PROGRAM IO_EXCHANGE
VAR
	WRITE_SINT			:	FB_EcCoESdoWrite	;
	sNetId              : 	T_AmsNetId := '10.4.6.84.7.1'; (* NetId of EtherCAT Master *)     
    nSlaveAddr_1        : 	UINT := 1003; (* Port Number of EtherCAT Slave *) 
	SDO_WRITE			:	STR_SDO	;
	WRITE_DATA_SINT		:	USINT;
	WRITE_EN_SINT		:	BOOL;
END_VAR

PLC_TO_UI();
UI_TO_PLC();

//************************HW-IO******************************************
//C02
		GV.NDI.	AV101_OPEN	:=	ECC.	CHAMBER_IN.		C02	[	1	];	//	AV101OPEN
		GV.NDI.	AV101_CLOSE	:=	ECC.	CHAMBER_IN.		C02	[	2	];	//	AV101CLOSE
		GV.NDI.	AV102_OPEN	:=	ECC.	CHAMBER_IN.		C02	[	3	];	//	AV102OPEN
	//	GV.NDI.	AV102_CLOSE	:=	ECC.	CHAMBER_IN.		C02	[	4	];	//	AV102CLOSE
	//	GV.NDI.	AV103_OPEN	:=									
	//	GV.NDI.	AV103_CLOSE	:=									
		GV.NDI.	AV104_OPEN	:=	ECC.	CHAMBER_IN.		C02	[	5	];	//	AV104OPEN
	//	GV.NDI.	AV104_CLOSE	:=	ECC.	CHAMBER_IN.		C02	[	6	];	//	AV104CLOSE
		GV.NDI.	AV105_OPEN	:=	ECC.	CHAMBER_IN.		C02	[	7	];	//	AV105OPEN
	//	GV.NDI.	AV105_CLOSE	:=	ECC.	CHAMBER_IN.		C02	[	8	];	//	AV105CLOSE
		GV.NDI.	AV106_OPEN	:=	ECC.	CHAMBER_IN.		C02	[	9	];	//	AV106OPEN
		GV.NDI.	AV106_CLOSE	:=	ECC.	CHAMBER_IN.		C02	[	10	];	//	AV106CLOSE
		GV.NDI.	CY1_OPEN	:=	ECC.	CHAMBER_IN.		C02	[	11	];	//	CY1 UP
		GV.NDI.	CY1_CLOSE	:=	ECC.	CHAMBER_IN.		C02	[	12	];	//	CY1 DOWN
		GV.NDI.	Lift_Pin_Middle1	:=	ECC.	CHAMBER_IN.		C02	[	13	];	//	CY1 Middle
		GV.NDI.	CY2_OPEN	:=	ECC.	CHAMBER_IN.		C02	[	14	];	//	CY2 UP						 
		GV.NDI.	CY2_CLOSE	:=	ECC.	CHAMBER_IN.		C02	[	15	];	//	CY2 DOWN
		GV.NDI.	Lift_Pin_Middle2	:=	ECC.	CHAMBER_IN.		C02	[	16	];	//	CY2 Middle								

//C03																											
		GV.NDI.	GV1_OPEN			:=	ECC.	CHAMBER_IN.		C03	[	1	];		//Slit Door Opened
		GV.NDI.	GV1_CLOSE			:=	ECC.	CHAMBER_IN.		C03	[	2	];		//Slit Door Closed
		GV.NDI.FL02B2				:=	ECC.	CHAMBER_IN.		C03	[	3	];		
		//							:=	ECC.	CHAMBER_IN.		C03	[	4	];		
		GV.NDI.FL03B2				:=	ECC.	CHAMBER_IN.		C03	[	5	];		
		//							:=	ECC.	CHAMBER_IN.		C03	[	6	];		
		GV.NDI.FL04B2				:=	ECC.	CHAMBER_IN.		C03	[	7	];		
		GV.NDI.Robot_Extend_TO_PM	:=	ECC.	CHAMBER_IN.		C03	[	8	];		//Robot Extend To PM
					//				:=	ECC.	CHAMBER_IN.		C03	[	9	];		
		GV.NDI.CDA_OK				:=	ECC.	CHAMBER_IN.		C03	[	10	];		
		GV.NDI.SYS_CDA_OK			:=	ECC.	CHAMBER_IN.		C03	[	11	];		//SYS CDA OK
		GV.NDI.SYS_N2_OK			:=	ECC.	CHAMBER_IN.		C03	[	12	];		//SYS N2 OK
		GV.NDI.TM_Lid_Closed		:=	ECC.	CHAMBER_IN.		C03	[	13	];		//TM Lid Closed
					//				:=	ECC.	CHAMBER_IN.		C03	[	14	];		
					//				:=	ECC.	CHAMBER_IN.		C03	[	15	];		//
					//				:=	ECC.	CHAMBER_IN.		C03	[	16	];		//

//C04
		GV.AI.	APC_Temp				:=			INT_TO_REAL(	ECC.	CHAMBER_IN.	C04	[	1	])/10;	//	SSR1	钟摆阀(E01)	TC01
		GV.AI.	Lid_Temp				:=			INT_TO_REAL(	ECC.	CHAMBER_IN.	C04	[	2	])/10;	//	SSR2	LID HEATER控温TC	(E02-E05) TC02
		GV.AI.	Lid_Temp_Monitor1		:=			INT_TO_REAL(	ECC.	CHAMBER_IN.	C04	[	3	])/10;	//	LID HEATER TC monitor	TC03
		GV.AI.	Lid_Temp_Monitor2		:=			INT_TO_REAL(	ECC.	CHAMBER_IN.	C04	[	4	])/10;	//	LID HEATER TC monitor	TC04
		GV.AI.	Chamber_Temp1			:=			INT_TO_REAL(	ECC.	CHAMBER_IN.	C04	[	5	])/10;	//	SSR3	CHAMBER HEATER 控温TC (E06,E07)	TC05
		GV.AI.	Chamber_Temp2			:=			INT_TO_REAL(	ECC.	CHAMBER_IN.	C04	[	6	])/10;	//	SSR4	CHAMBER HEATER 控温TC (E08,E09,E12,E13)	TC06
		GV.AI.	Chamber_Temp3			:=			INT_TO_REAL(	ECC.	CHAMBER_IN.	C04	[	7	])/10;	//	SSR5	CHAMBER HEATER 控温TC (E10,E11)			TC07
		GV.AI.	Stage_Temp1				:=			INT_TO_REAL(	ECC.	CHAMBER_IN.	C04	[	8	])/10;	//	CHILLER控温用(左侧内)	TC08

//C05		
		GV.AI.	Stage_Temp2				:=			INT_TO_REAL(	ECC.	CHAMBER_IN.	C05	[	1	])/10;	//	CHILLER控温用(左侧外)	TC09 
		GV.AI.	Stage_Temp3				:=			INT_TO_REAL(	ECC.	CHAMBER_IN.	C05	[	2	])/10;	//	CHILLER控温用(右侧内)	TC10
		GV.AI.	Stage_Temp4				:=			INT_TO_REAL(	ECC.	CHAMBER_IN.	C05	[	3	])/10;	//	CHILLER控温用(右侧外)	TC11
		GV.AI.	Chamber_Temp_Monitor	:=			INT_TO_REAL(	ECC.	CHAMBER_IN.	C05	[	4	])/10;	//	腔体底部监控用	TC12
		GV.AI.	Gate_Valve_Temp			:=			INT_TO_REAL(	ECC.	CHAMBER_IN.	C05	[	5	])/10;	//	SSR18	GATE VALVE控温用	E18 TC13
		GV.AI.	Gate_Valve_Temp_Monitor	:=			INT_TO_REAL(	ECC.	CHAMBER_IN.	C05	[	6	])/10;	//	GATE VALVE监控	TC14
										//			INT_TO_REAL(	ECC.	CHAMBER_IN.	C05	[	7	])/10;	//	
										//			INT_TO_REAL(	ECC.	CHAMBER_IN.	C05	[	8	])/10;	//	

//C06							
										//							ECC.	CHAMBER_IN.	C06	[	1	]);
										//							ECC.	CHAMBER_IN.	C06	[	2	]);
										//							ECC.	CHAMBER_IN.	C06	[	3	]);
										//							ECC.	CHAMBER_IN.	C06	[	4	]);

							
//C07											
		ECC.	CHAMBER_OUT.	C07	[	1	]	:=	TRUE;//GV_IL.TMP_PW_EN;//GV.TURBO_PUMP_POWER_ON							;	
		ECC.	CHAMBER_OUT.	C07	[	2	]	:=	GV_IL.HTR_APC_EN;//GV.PENDULUM_VALVE_HEATER_POWER_ON				;	
		ECC.	CHAMBER_OUT.	C07	[	3	]	:=	GV_IL.HTR_LID_EN;//GV.LID_HEATER_POWER_ON							;	
		ECC.	CHAMBER_OUT.	C07	[	4	]	:=	GV_IL.HTR_CHAMBER_EN;//GV.CHAMBER_HEATER_POWER_ON						;	
		ECC.	CHAMBER_OUT.	C07	[	5	]	:=	GV_IL.HTR_GAS_BOX_EN;//GV.IGS_HEATER_POWER_ON							;	
		ECC.	CHAMBER_OUT.	C07	[	6	]	:=	GV_IL.HTR_GAS_BOX_EN;//GV.TAPE_HEATER_POWER_ON							;	
		ECC.	CHAMBER_OUT.	C07	[	7	]	:=	GV_IL.HTR_FORLINE_EN;//GV.FORELINE_HEATER_POWER_ON						;	
		ECC.	CHAMBER_OUT.	C07	[	8	]	:=	GV_IL.HTR_GATE_VALVE_EN;//GV.GATE_VALVE_HEATER_POWER_ON					;	
	//	ECC.	CHAMBER_OUT.	C07	[	9	]	:=			;	
	//	ECC.	CHAMBER_OUT.	C07	[	10	]	:=			;	
	//	ECC.	CHAMBER_OUT.	C07	[	11	]	:=			;	
	//	ECC.	CHAMBER_OUT.	C07	[	12	]	:=			;	
		ECC.	CHAMBER_OUT.	C07	[	13	]	:=	GV.NDO.GV_Open_Enable		;	//Slit Door Open Enable
		ECC.	CHAMBER_OUT.	C07	[	14	]	:=	GV.NDO.GV_Close_Enable		;	//Slit Door Close Enable
		ECC.	CHAMBER_OUT.	C07	[	15	]	:=	GV.NDO.TM_Robot_Extend_Enable AND GV.NDI.CY1_OPEN AND GV.NDI.CY2_OPEN		;	//Robot Extend Enable
		ECC.	CHAMBER_OUT.	C07	[	16	]	;//:=			;	
												
//C08												
		ECC.	CHAMBER_OUT.	C08	[	1	]	:=	GV.LID_HEATER_SSR_ON[1]		;	//SSR02
	//	ECC.	CHAMBER_OUT.	C08	[	2	]	:=	GV.LID_HEATER_SSR_ON[2]		;	//SSR02
	//	ECC.	CHAMBER_OUT.	C08	[	3	]	:=	GV.LID_HEATER_SSR_ON[3]		;	//SSR02
	//	ECC.	CHAMBER_OUT.	C08	[	4	]	:=	GV.LID_HEATER_SSR_ON[4]		;	//SSR02
	//	ECC.	CHAMBER_OUT.	C08	[	5	]	:=								;	
	//	ECC.	CHAMBER_OUT.	C08	[	6	]	:=								;	
		ECC.	CHAMBER_OUT.	C08	[	7	]	:=	GV.CHAMBER_HEATER_SSR_ON[1]	;	//SSR03
		ECC.	CHAMBER_OUT.	C08	[	8	]	:=	GV.CHAMBER_HEATER_SSR_ON[2]	;	//SSR03
		ECC.	CHAMBER_OUT.	C08	[	9	]	:=	GV.CHAMBER_HEATER_SSR_ON[3]	;	//SSR04	
	//	ECC.	CHAMBER_OUT.	C08	[	10	]	:=	
		ECC.	CHAMBER_OUT.	C08	[	11	]	:=	GV.CHAMBER_HEATER_SSR_ON[4];	//SSR05
	//	ECC.	CHAMBER_OUT.	C08	[	12	]	:=	
		ECC.	CHAMBER_OUT.	C08	[	13	]	:=	
	//	ECC.	CHAMBER_OUT.	C08	[	14	]	:=	
	//	ECC.	CHAMBER_OUT.	C08	[	15	]	:=								;	
	//	ECC.	CHAMBER_OUT.	C08	[	16	]	:=								;	
												
//C09												
		ECC.	CHAMBER_OUT.	C09	[	1	]	:=	GV.FORELINE_HEATER_SSR_ON[1];	//SSR6	AV102 E33
		ECC.	CHAMBER_OUT.	C09	[	2	]	:=	GV.FORELINE_HEATER_SSR_ON[2];	//SSR7	AV101 E36
		ECC.	CHAMBER_OUT.	C09	[	3	]	:=	GV.FORELINE_HEATER_SSR_ON[3];	//SSR8	AV106	E38
		ECC.	CHAMBER_OUT.	C09	[	4	]	:=	GV.FORELINE_HEATER_SSR_ON[4];	//SSR9	BA01	
	//	ECC.	CHAMBER_OUT.	C09	[	5	]	:=								;	
	//	ECC.	CHAMBER_OUT.	C09	[	6	]	:=								;	
		ECC.	CHAMBER_OUT.	C09	[	7	]	:=	GV.GATE_VALVE_SSR_ON		;	//SSR18
	//	ECC.	CHAMBER_OUT.	C09	[	8	]	:=								;	
		ECC.	CHAMBER_OUT.	C09	[	9	]	:=	GV.PEN_VALVE_HEATER_SSR_ON	;	//SSR01
	//	ECC.	CHAMBER_OUT.	C09	[	10	]	:=								;	
		ECC.	CHAMBER_OUT.	C09	[	11	]	:=	GV.FORELINE_HEATER_SSR_ON[5];	//SSR10	VG103
		ECC.	CHAMBER_OUT.	C09	[	12	]	:=	GV.FORELINE_HEATER_SSR_ON[6];	//SSR11	EXHAUST1-6
		ECC.	CHAMBER_OUT.	C09	[	13	]	:=	GV.FORELINE_HEATER_SSR_ON[7];	//SSR12	EXHAUST7-8
		ECC.	CHAMBER_OUT.	C09	[	14	]	:=	GV.FORELINE_HEATER_SSR_ON[8];	//SSR13	
	//	ECC.	CHAMBER_OUT.	C09	[	15	]	:=								;	
	//	ECC.	CHAMBER_OUT.	C09	[	16	]	:=								;	
		
//C15
		GV.AI.VG103_Pipe_Temp			:=			INT_TO_REAL(	ECC.	CHAMBER_IN.	C15	[	1	])/10;	//	TC-03-A	SSR10	AV104+VG103_PIPE_1+VG103_PIPE_2
		GV.AI.BA01_Temp					:=			INT_TO_REAL(	ECC.	CHAMBER_IN.	C15	[	2	])/10;	//	TC-06-A	SSR09	BA101腔体侧+BA101
		GV.AI.VG101_Pipe_Temp			:=			INT_TO_REAL(	ECC.	CHAMBER_IN.	C15	[	3	])/10;	//	TC-07-A	SSR13	PS10+PS11
		GV.AI.Exhaust1_6_Temp			:=			INT_TO_REAL(	ECC.	CHAMBER_IN.	C15	[	4	])/10;	//	TC-29-A	SSR11	EXHAUST OUT1-6 E29-E32 E34-E35
		GV.AI.AV102_Temp				:=			INT_TO_REAL(	ECC.	CHAMBER_IN.	C15	[	5	])/10;	//	TC-33-A	SSR06	AV102
		GV.AI.AV101_Temp				:=			INT_TO_REAL(	ECC.	CHAMBER_IN.	C15	[	6	])/10;	//	TC-36-A	SSR07	AV101
		GV.AI.Exhaust7_8_Temp			:=			INT_TO_REAL(	ECC.	CHAMBER_IN.	C15	[	7	])/10;	//	TC-37-A	SSR12	EXHAUST7+8  E37+E39
		GV.AI.AV106_Temp				:=			INT_TO_REAL(	ECC.	CHAMBER_IN.	C15	[	8	])/10;	//	TC-38-A	SSR08	AV106
	

//C32												
		GV.AI.PG_PS1_VALUE	:=	(ECC.	IGS_IN.		C32	[	1	]*115/32767-15)*6.895;		
		GV.AI.PG_PS2_VALUE	:=	(ECC.	IGS_IN.		C32	[	2	]*115/32767-15)*6.895;		
		GV.AI.PG_PS3_VALUE	:=	(ECC.	IGS_IN.		C32	[	3	]*115/32767-15)*6.895;		
		GV.AI.PG_PS4_VALUE	:=	(ECC.	IGS_IN.		C32	[	4	]*115/32767-15)*6.895;		
												
//C33												
		GV.AI.PG_PS5_VALUE	:=	(ECC.	IGS_IN.		C33	[	1	]*75/32767-15)*6.895;		
		GV.AI.PG_PS6_VALUE	:=	(ECC.	IGS_IN.		C33	[	2	]*115/32767-15)*6.895;		
//		GV.AI.PG_PS7_VALUE	:=	(ECC.	IGS_IN.		C33	[	3	]*1015/32767-15)*6.895;		
//		GV.AI.PG_PS8_VALUE	:=	(ECC.	IGS_IN.		C33	[	4	]*1015/32767-15)*6.895;		
												
//C34												
//		GV.AI.PG_PS9_VALUE	:=	(ECC.	IGS_IN.		C34	[	1	]*1015/32767-15)*6.895;		
		GV.AI.PS1_VALUE		:=	(ECC.	IGS_IN.		C34	[	2	]*1015/32767-15)*6.895;		
		GV.AI.PS2_VALUE		:=	(ECC.	IGS_IN.		C34	[	3	]*1015/32767-15)*6.895;		
		GV.AI.MS1_VALUE		:=	(ECC.	IGS_IN.		C34	[	4	]*1015/32767-15)*6.895;		
												
//C35												
		GV.AI.GD01_VALUE	:=	ECC.	IGS_IN.		C35	[	1	];		
		GV.AI.GD02_VALUE	:=	ECC.	IGS_IN.		C35	[	2	];		
					//		:=	ECC.	IGS_IN.		C35	[	3	];		
					//		:=	ECC.	IGS_IN.		C35	[	4	];		
												
//C36												
		GV.NDI.	PG_PS1_Pressure_Switch_Up_Limit		:=	 ECC.	IGS_IN.		C36	[	1	];
		GV.NDI.	PG_PS1_Pressure_Switch_Down_Limit	:=	 ECC.	IGS_IN.		C36	[	2	];
		GV.NDI.	PG_PS2_Pressure_Switch_Up_Limit		:=	 ECC.	IGS_IN.		C36	[	3	];
		GV.NDI.	PG_PS2_Pressure_Switch_Down_Limit	:=	 ECC.	IGS_IN.		C36	[	4	];
		GV.NDI.	PG_PS3_Pressure_Switch_Up_Limit		:=	 ECC.	IGS_IN.		C36	[	5	];
		GV.NDI.	PG_PS3_Pressure_Switch_Down_Limit	:=	 ECC.	IGS_IN.		C36	[	6	];
		GV.NDI.	PG_PS4_Pressure_Switch_Up_Limit		:=	 ECC.	IGS_IN.		C36	[	7	];
		GV.NDI.	PG_PS4_Pressure_Switch_Down_Limit	:=	 ECC.	IGS_IN.		C36	[	8	];
		GV.NDI.	PG_PS5_Pressure_Switch_Up_Limit		:=	 ECC.	IGS_IN.		C36	[	9	];
		GV.NDI.	PG_PS5_Pressure_Switch_Down_Limit	:=	 ECC.	IGS_IN.		C36	[	10	];
		GV.NDI.	PG_PS6_Pressure_Switch_Up_Limit		:=	 ECC.	IGS_IN.		C36	[	11	];
		GV.NDI.	PG_PS6_Pressure_Switch_Down_Limit	:=	 ECC.	IGS_IN.		C36	[	12	];
//		GV.NDI.	PG_PS7_Pressure_Switch_Up_Limit		:=	 ECC.	IGS_IN.		C36	[	13	];
//		GV.NDI.	PG_PS7_Pressure_Switch_Down_Limit	:=	 ECC.	IGS_IN.		C36	[	14	];
//		GV.NDI.	PG_PS8_Pressure_Switch_Up_Limit		:=	 ECC.	IGS_IN.		C36	[	15	];
//		GV.NDI.	PG_PS8_Pressure_Switch_Down_Limit	:=	 ECC.	IGS_IN.		C36	[	16	];
											
//C37											
//		GV.NDI.	PG_PS9_Pressure_Switch_Up_Limit		:=	 ECC.	IGS_IN.		C37	[	1	];
//		GV.NDI.	PG_PS9_Pressure_Switch_Down_Limit	:=	 ECC.	IGS_IN.		C37	[	2	];
		//GV.NDI.	MS1_Pressure_Switch_Up_Limit		:=	 ECC.	IGS_IN.		C37	[	3	];
		GV.NDI.	MS1_ALM								:=	 ECC.	IGS_IN.		C37	[	4	];//QDP33P
		GV.NDI.	PS1_Pressure_Switch					:=	 ECC.	IGS_IN.		C37	[	5	];
		GV.NDI.	PS2_Pressure_Switch					:=	 ECC.	IGS_IN.		C37	[	6	];
											//		:=	ECC.	IGS_IN.		C37	[	7	];
											//		:=	ECC.	IGS_IN.		C37	[	8	];
											//		:=	ECC.	IGS_IN.		C37	[	9	];
											//		:=	ECC.	IGS_IN.		C37	[	10	];
											//		:=	ECC.	IGS_IN.		C37	[	11	];
											//		:=	ECC.	IGS_IN.		C37	[	12	];
											//		:=	ECC.	IGS_IN.		C37	[	13	];
											//		:=	ECC.	IGS_IN.		C37	[	14	];
											//		:=	ECC.	IGS_IN.		C37	[	15	];
											//		:=	ECC.	IGS_IN.		C37	[	16	];

(*												
//C38												
		GV.NDI.	GD001_ALM1							:=	ECC.	IGS_IN.		C38	[	1	];
		GV.NDI.	GD001_ALM2							:=	ECC.	IGS_IN.		C38	[	2	];
		GV.NDI.	GD002_ALM1							:=	ECC.	IGS_IN.		C38	[	3	];
		GV.NDI.	GD002_ALM2							:=	ECC.	IGS_IN.		C38	[	4	];

//C39																						
		GV.NDI.	GD_FAULT							:=	ECC.	IGS_IN.		C39	[	1	];
		GV.NDI.	MS1_Pressure_Switch_Up_Limit		:=	ECC.	IGS_IN.		C39	[	2	];
		GV.NDI.	MS1_Pressure_Switch_Down_Limit		:=	ECC.	IGS_IN.		C39	[	3	];
					//								:=	ECC.	IGS_IN.		C39	[	4	];
*)
//C40																							
		GV.AI.Tape_Temp1	:=	INT_TO_REAL(	ECC.	IGS_IN.	C40	[	1	])/10;	//	IGS 加热带			TC31	E31
		GV.AI.Tape_Temp2	:=	INT_TO_REAL(	ECC.	IGS_IN.	C40	[	2	])/10;	//	IGS 加热带			TC32	E32
		GV.AI.IGS_Temp1		:=	INT_TO_REAL(	ECC.	IGS_IN.	C40	[	3	])/10;	//	IGS BLOCK HEATER	TC33	E33 绿+ 红-
		GV.AI.IGS_Temp2		:=	INT_TO_REAL(	ECC.	IGS_IN.	C40	[	4	])/10;	//	IGS BLOCK HEATER	TC34	E34 绿+ 红-
		GV.AI.Tape_Temp3	:=	INT_TO_REAL(	ECC.	IGS_IN.	C40	[	5	])/10;	//	IGS 加热带	TC35	E35
						//	:=	INT_TO_REAL(	ECC.	IGS_IN.	C40	[	6	])/10;	//	IGS BLOCK HEATER	TC36	E36
						//	:=	INT_TO_REAL(	ECC.	IGS_IN.	C40	[	7	])/10;		
						//	:=	INT_TO_REAL(	ECC.	IGS_IN.	C40	[	8	])/10;		

//C42												
		ECC.	IGS_OUT.	C42	[	1	]	:=	GV.TAPE_HEATER_SSR_ON[1]	;	//SSR31	GAS BOX内+外延1
		ECC.	IGS_OUT.	C42	[	2	]	:=	GV.TAPE_HEATER_SSR_ON[2]	;	//SSR32	外延2+外延3
		ECC.	IGS_OUT.	C42	[	3	]	:=	GV.TAPE_HEATER_SSR_ON[3]	;	//SSR33	阀体
	//	ECC.	IGS_OUT.	C42	[	4	]	:=			;	
	//	ECC.	IGS_OUT.	C42	[	5	]	:=			;	
	//	ECC.	IGS_OUT.	C42	[	6	]	:=			;	
		ECC.	IGS_OUT.	C42	[	7	]	:=	GV.IGS_HEATER_SSR_ON[1]		;	//SSR35
		ECC.	IGS_OUT.	C42	[	8	]	:=	GV.IGS_HEATER_SSR_ON[2]		;	//SSR36
	//	ECC.	IGS_OUT.	C42	[	9	]	:=			;	
	//	ECC.	IGS_OUT.	C42	[	10	]	:=			;	
	//	ECC.	IGS_OUT.	C42	[	11	]	:=			;	
	//	ECC.	IGS_OUT.	C42	[	12	]	:=			;	
	//	ECC.	IGS_OUT.	C42	[	13	]	:=			;	
	//	ECC.	IGS_OUT.	C42	[	14	]	:=			;	
	//	ECC.	IGS_OUT.	C42	[	15	]	:=			;	
	//	ECC.	IGS_OUT.	C42	[	16	]	:=			;	
(*
//C43																								
		ECC.	IGS_OUT.	C43	[	1	]	:=	TRUE;//GV.VT03_POWER_ON		;	
	//	ECC.	IGS_OUT.	C43	[	2	]	:=			;	
	//	ECC.	IGS_OUT.	C43	[	3	]	:=			;	
	//	ECC.	IGS_OUT.	C43	[	4	]	:=			;	
*)

//MFC									
		GV.AI.	MFC1_Flow					:=	ECC.	MFC_PV	[	1	].Flow_Reading	;
		ECC.	MFC_SV	[	1	].Flow_SP	:=	GV.AO.	MFC1_Flow_Setpoint	;
		ECC.	MFC_SV	[	1	].Ramp_Time	:=	REAL_TO_UDINT(GV.AO.	MFC1_Rate_Setpoint)	;
		GV.AI.	MFC2_Flow					:=	ECC.	MFC_PV	[	2	].Flow_Reading	;
		ECC.	MFC_SV	[	2	].Flow_SP	:=	GV.AO.	MFC2_Flow_Setpoint	;
		ECC.	MFC_SV	[	2	].Ramp_Time	:=	REAL_TO_UDINT(GV.AO.	MFC2_Rate_Setpoint)	;
		GV.AI.	MFC3_Flow					:=	ECC.	MFC_PV	[	3	].Flow_Reading	;
		ECC.	MFC_SV	[	3	].Flow_SP	:=	GV.AO.	MFC3_Flow_Setpoint	;
		ECC.	MFC_SV	[	3	].Ramp_Time	:=	REAL_TO_UDINT(GV.AO.	MFC3_Rate_Setpoint)	;
(*		GV.AI.	MFC4_Flow					:=	ECC.	MFC_PV	[	4	].Flow_Reading	;
		ECC.	MFC_SV	[	4	].Flow_SP	:=	GV.AO.	MFC4_Flow_Setpoint	;
		ECC.	MFC_SV	[	4	].Ramp_Time	:=	REAL_TO_UDINT(GV.AO.	MFC4_Rate_Setpoint)	;
*)		GV.AI.	MFC5_Flow					:=	ECC.	MFC_PV	[	5	].Flow_Reading	;
		ECC.	MFC_SV	[	5	].Flow_SP	:=	GV.AO.	MFC5_Flow_Setpoint	;
		ECC.	MFC_SV	[	5	].Ramp_Time	:=	REAL_TO_UDINT(GV.AO.	MFC5_Rate_Setpoint)	;
		GV.AI.	MFC6_Flow					:=	ECC.	MFC_PV	[	6	].Flow_Reading	;
		ECC.	MFC_SV	[	6	].Flow_SP	:=	GV.AO.	MFC6_Flow_Setpoint	;
		ECC.	MFC_SV	[	6	].Ramp_Time	:=	REAL_TO_UDINT(GV.AO.	MFC6_Rate_Setpoint)	;
		GV.AI.	MFC7_Flow					:=	ECC.	MFC_PV	[	7	].Flow_Reading	;
		ECC.	MFC_SV	[	7	].Flow_SP	:=	GV.AO.	MFC7_Flow_Setpoint	;
		ECC.	MFC_SV	[	7	].Ramp_Time	:=	REAL_TO_UDINT(GV.AO.	MFC7_Rate_Setpoint)	;
	//	GV.AI.	MFC8_PV						:=	ECC.	MFC_PV	[	8	].Flow_Reading	;
	//	ECC.	MFC_SV	[	1	].Flow_SP	:=	GV.AO.	MFC8_Flow_Setpoint	;
	//	ECC.	MFC_SV	[	1	].Ramp_Time	:=	REAL_TO_UDINT(GV.AO.	MFC8_Rate_Setpoint)	;
	//	GV.AI.	MFC9_PV						:=	ECC.	MFC_PV	[	9	].Flow_Reading	;
	//	ECC.	MFC_SV	[	1	].Flow_SP	:=	GV.AO.	MFC9_Flow_Setpoint	;
	//	ECC.	MFC_SV	[	1	].Ramp_Time	:=	REAL_TO_UDINT(GV.AO.	MFC9_Rate_Setpoint)	;


	
//EV
		ECC.	EV1.	A.	0	:=	GV.	NDO.	GV101C;	//GATE VALVE CLOSE
		ECC.	EV1.	A.	1	:=	GV.	NDO. 	GV101O;	//GATE VALVE OPEN
	//	ECC.	EV1.	A.	2	:=	GV.	NDO.	
	//	ECC.	EV1.	A.	3	:=	GV.	NDO.	
		ECC.	EV1.	A.	4	:=	GV.	NDO.	AV110;	//PIN UP
		ECC.	EV1.	A.	5	:=	GV.	NDO.	AV109;	//PIN MIDDLE
		ECC.	EV1.	A.	6	:=	GV.	NDO.	AV103	AND GV_IL.AV103_EN;
		ECC.	EV1.	A.	7	:=	GV.	NDO.	AV104 	AND GV_IL.AV104_EN;	//VG103关断阀
		ECC.	EV1.	B.	0	:=	GV.	NDO.	AV101	AND GV_IL.AV101_EN;	//预抽阀
		ECC.	EV1.	B.	1	:=	GV.	NDO.	AV102	AND GV_IL.AV102_EN;	//分子泵前级阀
	//	ECC.	EV1.	B.	2	:=	GV.	NDO.		;
	//	ECC.	EV1.	B.	3	:=	GV.	NDO.		;
	//	ECC.	EV1.	B.	4	:=	GV.	NDO.		;
	//	ECC.	EV1.	B.	5	:=	GV.	NDO.		;
	//	ECC.	EV1.	B.	6	:=	GV.	NDO.		;
	//	ECC.	EV1.	B.	7	:=	GV.	NDO.		;

										
										
	//	ECC.	EV2.	A.	0	:=	GV.	NDO.	AV201	;
	//	ECC.	EV2.	A.	1	:=	GV.	NDO.	AC101	;
	//	ECC.	EV2.	A.	2	:=	GV.	NDO.	AC102	;
	//	ECC.	EV2.	A.	3	:=	GV.	NDO.	AC103	;
		ECC.	EV2.	A.	4	:=	GV.	NDO.	AV201	;	//进水管关断阀
	//	ECC.	EV2.	A.	5	:=	GV.	NDO.	AV202	;	//
		ECC.	EV2.	A.	6	:=	GV.	NDO.	AV107	;	//钟摆阀动作使能保持阀
		ECC.	EV2.	A.	7	:=	GV.	NDO.	AV108	;	//分子泵purge
		ECC.	EV2.	B.	0	:=	GV.	NDO.	AV105	AND GV_IL.AV105_EN;	//BA101关断阀
		ECC.	EV2.	B.	1	:=	GV.	NDO.	AV106	AND GV_IL.AV106_EN;	//酸排关断阀
	//	ECC.	EV2.	B.	2	:=	GV.	NDO.		;
	//	ECC.	EV2.	B.	3	:=	GV.	NDO.		;
	//	ECC.	EV2.	B.	4	:=	GV.	NDO.		;
	//	ECC.	EV2.	B.	5	:=	GV.	NDO.		;
	//	ECC.	EV2.	B.	6	:=	GV.	NDO.		;
	//	ECC.	EV2.	B.	7	:=	GV.	NDO.		;
	
										
//gas box内										
		ECC.	EV3.	A.	0	:=	GV.	NDO.	AV1	;	//
		ECC.	EV3.	A.	1	:=	GV.	NDO.	AV2	;
		ECC.	EV3.	A.	2	:=	GV.	NDO.	AV3	;
		ECC.	EV3.	A.	3	:=	GV.	NDO.	AV4	;
		ECC.	EV3.	A.	4	:=	GV.	NDO.	AV6	;
		ECC.	EV3.	A.	5	:=	GV.	NDO.	AV7	;
		ECC.	EV3.	A.	6	:=	GV.	NDO.	AV9	;
		ECC.	EV3.	A.	7	:=	GV.	NDO.	AV10;
		ECC.	EV3.	B.	0	:=	GV.	NDO.	AV11;
		ECC.	EV3.	B.	1	:=	GV.	NDO.	AV12;
		ECC.	EV3.	B.	2	:=	GV.	NDO.	AV13;
		ECC.	EV3.	B.	3	:=	GV.	NDO.	AV14;
		ECC.	EV3.	B.	4	:=	GV.	NDO.	AV16;
		ECC.	EV3.	B.	5	:=	GV.	NDO.	AV17;
		ECC.	EV3.	B.	6	:=	GV.	NDO.	AV19;
		ECC.	EV3.	B.	7	:=	GV.	NDO.	AV20;
		ECC.	EV3.	C.	0	:=	GV.	NDO.	AV22;
		ECC.	EV3.	C.	1	:=	GV.	NDO.	AV23;
		ECC.	EV3.	C.	2	:=	GV.	NDO.	AV25;
		ECC.	EV3.	C.	3	:=	GV.	NDO.	AV26;
		ECC.	EV3.	C.	4	:=	GV.	NDO.	AV27;
	//	ECC.	EV3.	C.	5	:=	GV.	NDO.		;
	//	ECC.	EV3.	C.	6	:=	GV.	NDO.		;
	//	ECC.	EV3.	C.	7	:=	GV.	NDO.		;
	//	ECC.	EV3.	D.	0	:=	GV.	NDO.		;
	//	ECC.	EV3.	D.	1	:=	GV.	NDO.		;
	//	ECC.	EV3.	D.	2	:=	GV.	NDO.		;
	//	ECC.	EV3.	D.	3	:=	GV.	NDO.		;
	//	ECC.	EV3.	D.	4	:=	GV.	NDO.		;
	//	ECC.	EV3.	D.	5	:=	GV.	NDO.		;
	//	ECC.	EV3.	D.	6	:=	GV.	NDO.		;
	//	ECC.	EV3.	D.	7	:=	GV.	NDO.		;
										
										
//gas box内										
	//	ECC.	EV4.	A.	0	:=	GV.	NDO.	AV5	;
		ECC.	EV4.	A.	1	:=	GV.	NDO.	AV5	;
	//	ECC.	EV4.	A.	2	:=	GV.	NDO.	AV8	;
		ECC.	EV4.	A.	3	:=	GV.	NDO.	AV8	;
	//	ECC.	EV4.	A.	4	:=	GV.	NDO.	AV15	;
		ECC.	EV4.	A.	5	:=	GV.	NDO.	AV15	;
	//	ECC.	EV4.	A.	6	:=	GV.	NDO.	AV18	;
		ECC.	EV4.	A.	7	:=	GV.	NDO.	AV18	;
	//	ECC.	EV4.	B.	0	:=	GV.	NDO.	AV21	;
		ECC.	EV4.	B.	1	:=	GV.	NDO.	AV21	;
	//	ECC.	EV4.	B.	2	:=	GV.	NDO.	AV24	;
		ECC.	EV4.	B.	3	:=	GV.	NDO.	AV24	;
	//	ECC.	EV4.	B.	4	:=	GV.	NDO.		;
	//	ECC.	EV4.	B.	5	:=	GV.	NDO.		;
	//	ECC.	EV4.	B.	6	:=	GV.	NDO.		;
	//	ECC.	EV4.	B.	7	:=	GV.	NDO.		;
	




//APC											
	GV.	AI.	APC.	ACTUAL_PRESSURE					:=	ECC.			APC_PV.Actual_Pressure	*100/133.3*1000;	
	GV.	AI.	APC.	Pressure_Sensor_1				:=	ECC.			APC_PV.Pressure_Sensor_1	*100/133.3*1000;	
	GV.	AI.	APC.	Pressure_Sensor_2				:=	ECC.			APC_PV.Pressure_Sensor_2	*100/133.3*1000;	
	GV.	AI.	APC.	ACTUAL_POSITION					:=	ECC.			APC_PV.Actual_Position	;	
	GV.	AI.	APC.	CONTROL_MODE					:=	ECC.			APC_PV.Control_Mode	;	
	GV.	AI.	APC.	ERROR_NUMBER					:=	ECC.			APC_PV.ERROR_NUMBER	;	
	GV.	AI.	APC.	General_Status					:=	ECC.			APC_PV.General_Status	;	
	GV.	AI.	APC.	GENERAL_WARNINGS				:=	ECC.			APC_PV.General_Warnings	;	
	GV.	AI.	APC.	Extended_Warnings				:=	ECC.			APC_PV.Extended_Warnings	;	
	ECC.	APC_SV.Target_Pressure					:=	GV.	AO.	APC.	TARGET_PRESSURE*0.1333/100	;	
	ECC.	APC_SV.Target_Position					:=	GV.	AO.	APC.	TARGET_POSITION	;	
	ECC.	APC_SV.Pressure_Input_Digital_Sensor_1	:=	GV.	AO.	APC.	Pressure_Input_Digital_Sensor_1	;	//E-therCAT通讯传送过来的sensor值1
	ECC.	APC_SV.Pressure_Input_Digital_Sensor_2	:=	GV.	AO.	APC.	Pressure_Input_Digital_Sensor_2	;	//E-therCAT通讯传送过来的sensor值2
	ECC.	APC_SV.Control_Mode						:=	GV.	AO.	APC.	CONTROL_MODE	;	
	ECC.	APC_SV.General_Control_Setpoint			:=	GV.	AO.	APC.	General_Control_Setpoint	;		(*Bit 0: Zero 
										 																	  BIT 1: NOT used 
																											  Bit 2: Ping Pong TX Bit
																											  Bit 3: Not Used
																											  Bit 4: Access Mode Locked (VAT使用手册P72)
																											  Bit 5-15: Not Used
																											*)
	ECC.	APC_SV.Pressure_Ramp_Time				:=	GV.	AO.	APC.	PRESSURE_RAMP_TIME	;	
	
	IF GV.	AO.	APC.	TARGET_PRESSURE>=1000
		THEN 
			ECC.APC_SV.Bank_Sel:=1;
		ELSIF
			GV.	AO.	APC.	TARGET_PRESSURE<1000 AND GV.	AO.	APC.	TARGET_PRESSURE>=100
		THEN 
			ECC.APC_SV.Bank_Sel:=2;
		ELSIF
			GV.	AO.	APC.	TARGET_PRESSURE<100
		THEN
			ECC.APC_SV.Bank_Sel:=3;
	END_IF
	
	IF ECC.	APC_SV.Control_Mode=7 AND ECC.APC_PV.Control_Mode<>7 THEN
		WRITE_EN_SINT:=TRUE;
		ELSE		
		WRITE_EN_SINT:=FALSE;
	END_IF
	
	WRITE_DATA_SINT:=ECC.APC_SV.Bank_Sel;
	SDO_WRITE.Index:=UINT#16#2350;
	SDO_WRITE.Subindex:=USINT#16#03;
	
	
	WRITE_SINT(
		sNetId:= sNetId, 						//主站IP地址, 
		nSlaveAddr:= nSlaveAddr_1, 				//从站端口
		nSubIndex:= USINT_TO_BYTE(SDO_WRITE.Subindex),	//SubIndex
		nIndex:= UINT_TO_WORD(SDO_WRITE.Index), 		//Index
		pSrcBuf:= ADR(WRITE_DATA_SINT), 
		cbBufLen:= SIZEOF(WRITE_DATA_SINT), 
		bExecute:= WRITE_EN_SINT, 
		//tTimeout:= T#200MS, 
		bBusy=> , 
		bError=> , 
		nErrId=> );	
											
//TMP											
	GV.	AI.	TMP.	ROTATION						:=	ECC.			TURBO_PV.Rotation	;	//1:ROTATING,0:NOT ROTATING
	GV.	AI.	TMP.	NORMAL							:=	ECC.			TURBO_PV.Normal	;		//1:NORMAL,0:UNNORMAL
	GV.	AI.	TMP.	ACCELERATION					:=	ECC.			TURBO_PV.Acceleration	;	
	GV.	AI.	TMP.	Deceleration_Includes_Braking	:=	ECC.			TURBO_PV.Deceleration_Includes_Braking	;	
	GV.	AI.	TMP.	REMOTE_LOCAL					:=	ECC.			TURBO_PV.Remote_Local	;	//1:LOCAL.E-CAT CONTROL DISABLED,0:REMOTE.E-CAT CONTROL ENABLED
	GV.	AI.	TMP.	Turbo_Low_Speed					:=	ECC.			TURBO_PV.Turbo_Low_Speed	;	
	GV.	AI.	TMP.	ALARM							:=	ECC.		TURBO_PV.Alarm	;	
	GV.	AI.	TMP.	WARNING							:=	ECC.		TURBO_PV.Warning	;	
	GV.	AI.	TMP.	Turbo_Speed						:=	REAL_TO_INT(ECC.TURBO_PV.Turbo_Speed*32.5	);	//0.1[%],1000(100.0%):RATED SPEED,0(0.0%):NO RATATION
	GV.	AI.	TMP.	Turbo_Current					:=	ECC.			TURBO_PV.Turbo_Current	;	//0.1A
	GV.	AI.	TMP.	Turbo_pump_temperature			:=	ECC.			TURBO_PV.Turbo_pump_temperature	;	//1[℃]
	//GV.	AI.	TMP.	VibrationH					:=	ECC.			TURBO_PV.VibrationH	;	
	//GV.	AI.	TMP.	VibrationB					:=	ECC.			TURBO_PV.VibrationB	;	
	//GV.	AI.	TMP.	VibrationZ					:=	ECC.			TURBO_PV.VibrationZ	;	
	ECC.			TURBO_SV.Turbo_Start_Stop		:=	GV.	AO.	TMP.	Turbo_Start_Stop	;	//1:START,0:STOP
	ECC.			TURBO_SV.Turbo_Reset_Alarm		:=	GV.	AO.	TMP.	Turbo_Reset_Alarm	;	//1:RESET ALARM,0:NO ACTION
	ECC.			TURBO_SV.Turbo_Low_Speed		:=	GV.	AO.	TMP.	Turbo_Low_Speed	;		//1:LOW SPEED MODE ON,0:OFF
	
//PG PS
	GV.AI.VG103_Pressure		:=	ECC.	VG103_PV.Sensor_Value1	/133.3	*1000					;
											
	GV.AI.VG101_Pressure		:=	ECC.	VG101_PV.Sensor_Value1	/133.3	*1000					;
											
	GV.AI.VG102_Pressure		:=	ECC.	VG102_PV.Sensor_Value1	/133.3	*1000					;
											
	GV.AI.BA1_Pressure			:=	ECC.	BA1_PV.Combination_Gauge_Active_Value_Module_1	/133.3	;
											
	GV.AI.VG104_Pressure		:=	ECC.	VG104_PV.Sensor_Value1	/133.3	*1000					;

//CHILLER
	GV.	AI.CHILLER1_TEMP_PV						:=	UINT_TO_REAL(	ECC.	CHILLER1_PV.Module2_Word[1]	)/10	;	//有符号整数，-50.0 to 150.0℃ = FE0Ch to 05DCh ,0.1℃/dig
	GV.	AI.CHILLER1_DI_PV						:=	UINT_TO_REAL(	ECC.	CHILLER1_PV.Module2_Word[2]	)	;	//	0.0 to 20.0M-ohm = 0000h to 00C8h ,0.1M-ohm/dig
	GV.	AI.CHILLER1_FLOW_PV						:=	UINT_TO_REAL(	ECC.	CHILLER1_PV.Module2_Word[3]	)	;	//	0.0 to 150.0LPM = 0000h to 05DCh 0.1LPM/dig
	GV.	AI.CHILLER1_PRESS_PV					:=	UINT_TO_REAL(	ECC.	CHILLER1_PV.Module2_Word[4]	)	;	//	0.00 to 2.00MPa = 0h to C8h 0.01MP/dig
	ECC.CHILLER1_SV.Module2_Word[1]				:=	REAL_TO_UINT(	GV.		AO.Chiller1_On					)	;	//CHILLER1 ON
	ECC.CHILLER1_SV.Module2_Word[2]				:=	REAL_TO_UINT(	GV.		AO.Chiller_Temp1_SV	*10			)	;	// -20.0 to 90.0℃= FF38h to 384h 0.1℃/dig
	ECC.CHILLER1_SV.Module2_Word[3]				:=	INT_TO_UINT(	ECC.	CHAMBER_IN.	C04	[	8	]		)	;	// Stage温度反馈给chiller
	
	GV.	AI.CHILLER2_TEMP_PV						:=	UINT_TO_REAL(	ECC.	CHILLER2_PV.Module2_Word[1]	)/10	;	//有符号整数，-50.0 to 150.0℃ = FE0Ch to 05DCh ,0.1℃/dig
	GV.	AI.CHILLER2_DI_PV						:=	UINT_TO_REAL(	ECC.	CHILLER2_PV.Module2_Word[2]	)	;	//	0.0 to 20.0M-ohm = 0000h to 00C8h ,0.1M-ohm/dig
	GV.	AI.CHILLER2_FLOW_PV						:=	UINT_TO_REAL(	ECC.	CHILLER2_PV.Module2_Word[3]	)	;	//	0.0 to 150.0LPM = 0000h to 05DCh 0.1LPM/dig
	GV.	AI.CHILLER2_PRESS_PV					:=	UINT_TO_REAL(	ECC.	CHILLER2_PV.Module2_Word[4]	)	;	//	0.00 to 2.00MPa = 0h to C8h 0.01MP/dig
	ECC.CHILLER2_SV.Module2_Word[1]				:=	REAL_TO_UINT(	GV.		AO.Chiller2_On					)	;	//CHILLER1 ON
	ECC.CHILLER2_SV.Module2_Word[2]				:=	REAL_TO_UINT(	GV.		AO.Chiller_Temp2_SV	*10			)	;	// -20.0 to 90.0℃= FF38h to 384h 0.1℃/dig
	ECC.CHILLER2_SV.Module2_Word[3]				:=	INT_TO_UINT(	ECC.	CHAMBER_IN.	C05	[	2	]		)	;	// Stage温度反馈给chiller

ACTION PLC_TO_UI:
PM.HeartBeat:=UI.HeartBeat;
PM.NDI:=GV.NDI;
PM.AI:=GV.AI;
GV.NDI.	AV1	:=GV.NDO.	AV1	;
GV.NDI.	AV2	:=GV.NDO.	AV2	;
GV.NDI.	AV3	:=GV.NDO.	AV3	;
GV.NDI.	AV4	:=GV.NDO.	AV4	;
GV.NDI.	AV5	:=GV.NDO.	AV5	;
GV.NDI.	AV6	:=GV.NDO.	AV6	;
GV.NDI.	AV7	:=GV.NDO.	AV7	;
GV.NDI.	AV8	:=GV.NDO.	AV8	;
GV.NDI.	AV9	:=GV.NDO.	AV9	;
GV.NDI.	AV10	:=GV.NDO.	AV10	;
GV.NDI.	AV11	:=GV.NDO.	AV11	;
GV.NDI.	AV12	:=GV.NDO.	AV12	;
GV.NDI.	AV13	:=GV.NDO.	AV13	;
GV.NDI.	AV14	:=GV.NDO.	AV14	;
GV.NDI.	AV15	:=GV.NDO.	AV15	;
GV.NDI.	AV16	:=GV.NDO.	AV16	;
GV.NDI.	AV17	:=GV.NDO.	AV17	;
GV.NDI.	AV18	:=GV.NDO.	AV18	;
GV.NDI.	AV19	:=GV.NDO.	AV19	;
GV.NDI.	AV20	:=GV.NDO.	AV20	;
GV.NDI.	AV21	:=GV.NDO.	AV21	;
GV.NDI.	AV22	:=GV.NDO.	AV22	;
GV.NDI.	AV23	:=GV.NDO.	AV23	;
GV.NDI.	AV24	:=GV.NDO.	AV24	;
GV.NDI.	AV25	:=GV.NDO.	AV25	;
GV.NDI.	AV26	:=GV.NDO.	AV26	;
GV.NDI.	AV27	:=GV.NDO.	AV27	;
END_ACTION

ACTION UI_TO_PLC:

	
//CONFIG
	GV.PMConfig:=UI.PMConfig;

	
	GV.Chiller:=UI.Chiller;
	GV.InnerChiller:=UI.InnerChiller;
	GV.OuterChiller:=UI.OuterChiller;
	GV.TopChiller:=UI.TopChiller;
	
	GV.DryPump:=UI.DryPump;
	
	GV.Mfcgas1:=UI.Mfcgas1;
	GV.Mfcgas2:=UI.Mfcgas2;
	GV.Mfcgas3:=UI.Mfcgas3;
	GV.Mfcgas4:=UI.Mfcgas4;
	GV.Mfcgas5:=UI.Mfcgas5;
	GV.Mfcgas6:=UI.Mfcgas6;
	GV.Mfcgas7:=UI.Mfcgas7;
	GV.Mfcgas8:=UI.Mfcgas8;
	GV.Mfcgas9:=UI.Mfcgas9;
	GV.Mfcgas10:=UI.Mfcgas10;
	GV.Mfcgas11:=UI.Mfcgas11;
	GV.Mfcgas12:=UI.Mfcgas12;
	GV.MfcN2:=UI.MfcN2;
	GV.MfcHe:=UI.MfcHe;
	
	GV.Pump:=UI.Pump;
	
	GV.Purge:=UI.Purge;
	
	GV.PendulumHeater:=UI.PendulumHeater;
	GV.LidHeater:=UI.LidHeater;
	GV.ChamberHeater:=UI.ChamberHeater;
	GV.IGSHeater:=UI.IGSHeater;
	GV.TapeHeater:=UI.TapeHeater;
	GV.ForelineHeater:=UI.ForelineHeater;


	
	GV.PendulumValve:=UI.PendulumValve;


	GV.ChamberHeater:=UI.ChamberHeater;
	GV.ChamberHeater:=UI.ChamberHeater;

//Status	
	GV.AO.	AV102_Temp_SV								:=	UI.AO.	AV102_Temp_SV			;
	GV.AO.	AV101_Temp_SV								:=	UI.AO.	AV101_Temp_SV			;
	GV.AO.	AV106_Temp_SV								:=	UI.AO.	AV106_Temp_SV			;
	GV.AO.	BA01_Temp_SV								:=	UI.AO.	BA01_Temp_SV			;
	GV.AO.	VG103_Pipe_Temp_SV							:=	UI.AO.	VG103_Pipe_Temp_SV		;
	GV.AO.	Exhaust1_6_Temp_SV							:=	UI.AO.	Exhaust1_6_Temp_SV		;
	GV.AO.	Exhaust7_8_Temp_SV							:=	UI.AO.	Exhaust7_8_Temp_SV		;
	GV.AO.	VG101_Pipe_Temp_SV							:=	UI.AO.	VG101_Pipe_Temp_SV		;
	GV.AO.	Gate_Valve_Temp_SV							:=	UI.AO.	Gate_Valve_Temp_SV		;
	GV.AO.	APC_Temp_SV									:=	UI.AO.	APC_Temp_SV		;
//	GV.AO.	TMP_Temp_SV									:=	UI.AO.	TMP_Temp_SV		;
	GV.AO.	Tape_Temp1_SV								:=	UI.AO.	Tape_Temp1_SV		;
	GV.AO.	Tape_Temp2_SV								:=	UI.AO.	Tape_Temp2_SV		;
	GV.AO.	Tape_Temp3_SV								:=	UI.AO.	Tape_Temp3_SV		;
	GV.AO.	IGS_Temp1_SV								:=	UI.AO.	IGS_Temp1_SV		;
	GV.AO.	IGS_Temp2_SV								:=	UI.AO.	IGS_Temp2_SV		;
	GV.AO.	Chiller_Temp1_SV							:=	UI.AO.	Chiller_Temp1_SV		;
	GV.AO.	Chiller_Temp2_SV							:=	UI.AO.	Chiller_Temp2_SV		;
	GV.AO.	Chiller1_On									:=	UI.AO.	Chiller1_On			;
	GV.AO.	Chiller2_On									:=	UI.AO.	Chiller2_On			;
	GV.AO.	TMP.	Turbo_Start_Stop					:=	UI.AO.	TMP.	Turbo_Start_Stop	;
	GV.AO.	TMP.	Turbo_Reset_Alarm					:=	UI.AO.	TMP.	Turbo_Reset_Alarm	;
	GV.AO.	TMP.	Turbo_Low_Speed						:=	UI.AO.	TMP.	Turbo_Low_Speed	;
	
	GV.NDO.AV104:=UI.NDO.AV104;
	GV.NDO.AV105:=UI.NDO.AV105;
	
	IF NOT MAIN.Process_EN THEN	
	GV.NDO	.	AV101	:=	UI.NDO	.	AV101	AND 	GV_IL.	AV101_EN;
	GV.NDO	.	AV102	:=	UI.NDO	.	AV102	AND 	GV_IL.	AV102_EN;
	GV.NDO	.	AV103	:=	UI.NDO	.	AV103	AND 	GV_IL.	AV103_EN;
	GV.NDO	.	AV104	:=	UI.NDO	.	AV104	AND 	GV_IL.	AV104_EN;
	GV.NDO	.	AV105	:=	UI.NDO	.	AV105	AND 	GV_IL.	AV105_EN;
	GV.NDO	.	AV106	:=	UI.NDO	.	AV106	AND 	GV_IL.	AV106_EN;
	GV.NDO	.	AV107	:=	UI.NDO	.	AV107				;
	GV.NDO	.	AV108	:=	UI.NDO	.	AV108				;
	GV.NDO	.	AV109	:=	UI.NDO	.	AV109				;
	GV.NDO	.	AV110	:=	UI.NDO	.	AV110				;
	GV.NDO	.	GV101C	:=	UI.NDO	.	GV101C				;
	GV.NDO	.	GV101O	:=	UI.NDO	.	GV101O				;
	GV.NDO	.	AV201	:=	UI.NDO	.	AV201				;
	GV.NDO	.	AV202	:=	UI.NDO	.	AV202				;
	GV.NDO	.	AC101	:=	UI.NDO	.	AC101				;
	GV.NDO	.	AC102	:=	UI.NDO	.	AC102				;
	GV.NDO	.	AC103	:=	UI.NDO	.	AC103				;
	GV.NDO	.	AC104	:=	UI.NDO	.	AC104				;
	GV.NDO	.	AC105	:=	UI.NDO	.	AC105				;
	GV.NDO	.	AC106	:=	UI.NDO	.	AC106				;
	GV.NDO	.	AV1	:=	UI.NDO	.	AV1	AND 	GV_IL.	AV1_EN	;
	GV.NDO	.	AV2	:=	UI.NDO	.	AV2	AND 	GV_IL.	AV2_EN	;
	GV.NDO	.	AV3	:=	UI.NDO	.	AV3	AND 	GV_IL.	AV3_EN	;
	GV.NDO	.	AV4	:=	UI.NDO	.	AV4	AND 	GV_IL.	AV4_EN	;
	GV.NDO	.	AV6	:=	UI.NDO	.	AV6	AND 	GV_IL.	AV6_EN	;
	GV.NDO	.	AV7	:=	UI.NDO	.	AV7	AND 	GV_IL.	AV7_EN	;
	GV.NDO	.	AV9	:=	UI.NDO	.	AV9	AND 	GV_IL.	AV9_EN	;
	GV.NDO	.	AV10	:=	UI.NDO	.	AV10	AND 	GV_IL.	AV10_EN	;
	GV.NDO	.	AV11	:=	UI.NDO	.	AV11	AND 	GV_IL.	AV11_EN	;
	GV.NDO	.	AV12	:=	UI.NDO	.	AV12	AND 	GV_IL.	AV12_EN	;
	GV.NDO	.	AV13	:=	UI.NDO	.	AV13	AND 	GV_IL.	AV13_EN	;
	GV.NDO	.	AV14	:=	UI.NDO	.	AV14	AND 	GV_IL.	AV14_EN	;
	GV.NDO	.	AV16	:=	UI.NDO	.	AV16	AND 	GV_IL.	AV16_EN	;
	GV.NDO	.	AV17	:=	UI.NDO	.	AV17	AND 	GV_IL.	AV17_EN	;
	GV.NDO	.	AV19	:=	UI.NDO	.	AV19	AND 	GV_IL.	AV19_EN	;
	GV.NDO	.	AV20	:=	UI.NDO	.	AV20	AND 	GV_IL.	AV20_EN	;
	GV.NDO	.	AV22	:=	UI.NDO	.	AV22	AND 	GV_IL.	AV22_EN	;
	GV.NDO	.	AV23	:=	UI.NDO	.	AV23	AND 	GV_IL.	AV23_EN	;
	GV.NDO	.	AV25	:=	UI.NDO	.	AV25	AND 	GV_IL.	AV25_EN	;
	GV.NDO	.	AV26	:=	UI.NDO	.	AV26	AND 	GV_IL.	AV26_EN	;
	GV.NDO	.	AV27	:=	UI.NDO	.	AV27	AND 	GV_IL.	AV27_EN	;
	GV.NDO	.	AV5	:=	UI.NDO	.	AV5	AND 	GV_IL.	AV5_EN	;
	GV.NDO	.	AV8	:=	UI.NDO	.	AV8	AND 	GV_IL.	AV8_EN	;
	GV.NDO	.	AV15	:=	UI.NDO	.	AV15	AND 	GV_IL.	AV15_EN	;
	GV.NDO	.	AV18	:=	UI.NDO	.	AV18	AND 	GV_IL.	AV18_EN	;
	GV.NDO	.	AV21	:=	UI.NDO	.	AV21	AND 	GV_IL.	AV21_EN	;
	GV.NDO	.	AV24	:=	UI.NDO	.	AV24	AND 	GV_IL.	AV24_EN	;
	GV.NDO	.	MaualEndStep	:=	UI.NDO	.	MaualEndStep				;


	GV.AO.	LID_Temp_SV		:=	UI.AO.	LID_Temp_SV		;

	GV.AO.	Chamber_Temp1_SV	:=	UI.AO.	Chamber_Temp1_SV		;
	GV.AO.	Chamber_Temp2_SV	:=	UI.AO.	Chamber_Temp2_SV		;
	GV.AO.	Chamber_Temp3_SV	:=	UI.AO.	Chamber_Temp3_SV		;

	GV.AO.	MFC1_Flow_Setpoint	:=	UI.AO.	MFC1_Flow_Setpoint		;
	GV.AO.	MFC1_Rate_Setpoint	:=	UI.AO.	MFC1_Rate_Setpoint		;
	GV.AO.	MFC2_Flow_Setpoint	:=	UI.AO.	MFC2_Flow_Setpoint		;
	GV.AO.	MFC2_Rate_Setpoint	:=	UI.AO.	MFC2_Rate_Setpoint		;
	GV.AO.	MFC3_Flow_Setpoint	:=	UI.AO.	MFC3_Flow_Setpoint		;
	GV.AO.	MFC3_Rate_Setpoint	:=	UI.AO.	MFC3_Rate_Setpoint		;
//	GV.AO.	MFC4_Flow_Setpoint	:=	UI.AO.	MFC4_Flow_Setpoint		;
//	GV.AO.	MFC4_Rate_Setpoint	:=	UI.AO.	MFC4_Rate_Setpoint		;
	GV.AO.	MFC5_Flow_Setpoint	:=	UI.AO.	MFC5_Flow_Setpoint		;
	GV.AO.	MFC5_Rate_Setpoint	:=	UI.AO.	MFC5_Rate_Setpoint		;
	GV.AO.	MFC6_Flow_Setpoint	:=	UI.AO.	MFC6_Flow_Setpoint		;
	GV.AO.	MFC6_Rate_Setpoint	:=	UI.AO.	MFC6_Rate_Setpoint		;
	GV.AO.	MFC7_Flow_Setpoint	:=	UI.AO.	MFC7_Flow_Setpoint		;
	GV.AO.	MFC7_Rate_Setpoint	:=	UI.AO.	MFC7_Rate_Setpoint		;
	GV.AO.	Stage_Temp1_SV		:=	UI.AO.	Stage_Temp1_SV		;
	GV.AO.	Stage_Temp2_SV		:=	UI.AO.	Stage_Temp2_SV		;
	GV.AO.	APC.	Target_Pressure	:=	UI.AO.	APC.	Target_Pressure	;
	GV.AO.	APC.	Target_Position	:=	UI.AO.	APC.	Target_Position	;
	//GV.AO.	APC.	Pressure_Input_Digital_Sensor_1	:=	UI.AO.	APC.	Pressure_Input_Digital_Sensor_1	;
	//GV.AO.	APC.	Pressure_Input_Digital_Sensor_2	:=	UI.AO.	APC.	Pressure_Input_Digital_Sensor_2	;
	IF GV_IL.APC_EN THEN 
		GV.AO.	APC.	Control_Mode	:=	UI.AO.	APC.	Control_Mode	;
	ELSE 
		GV.AO.	APC.	Control_Mode	:=	3	;
	END_IF
	GV.AO.	APC.	General_Control_Setpoint	:=	UI.AO.	APC.	General_Control_Setpoint	;
	GV.AO.	APC.	Pressure_Ramp_Time	:=	UI.AO.	APC.	Pressure_Ramp_Time	;
	GV.NDO.GV_Open_Enable:=NOT MAIN.Process_EN;
	GV.NDO.GV_Close_Enable:=NOT MAIN.Process_EN;
	GV.NDO.TM_Robot_Extend_Enable:=UI.NDO.TM_Robot_Extend_Enable;
	END_IF

//RECIPE
	GV.Step_Num:=UI.Step_Num;
	GV.SetpArray:=UI.SetpArray;
	
	GV.Process_Start:=UI.Process_Start;
	GV.Process_Stop:=UI.Process_Stop;
END_ACTION

END_PROGRAM
